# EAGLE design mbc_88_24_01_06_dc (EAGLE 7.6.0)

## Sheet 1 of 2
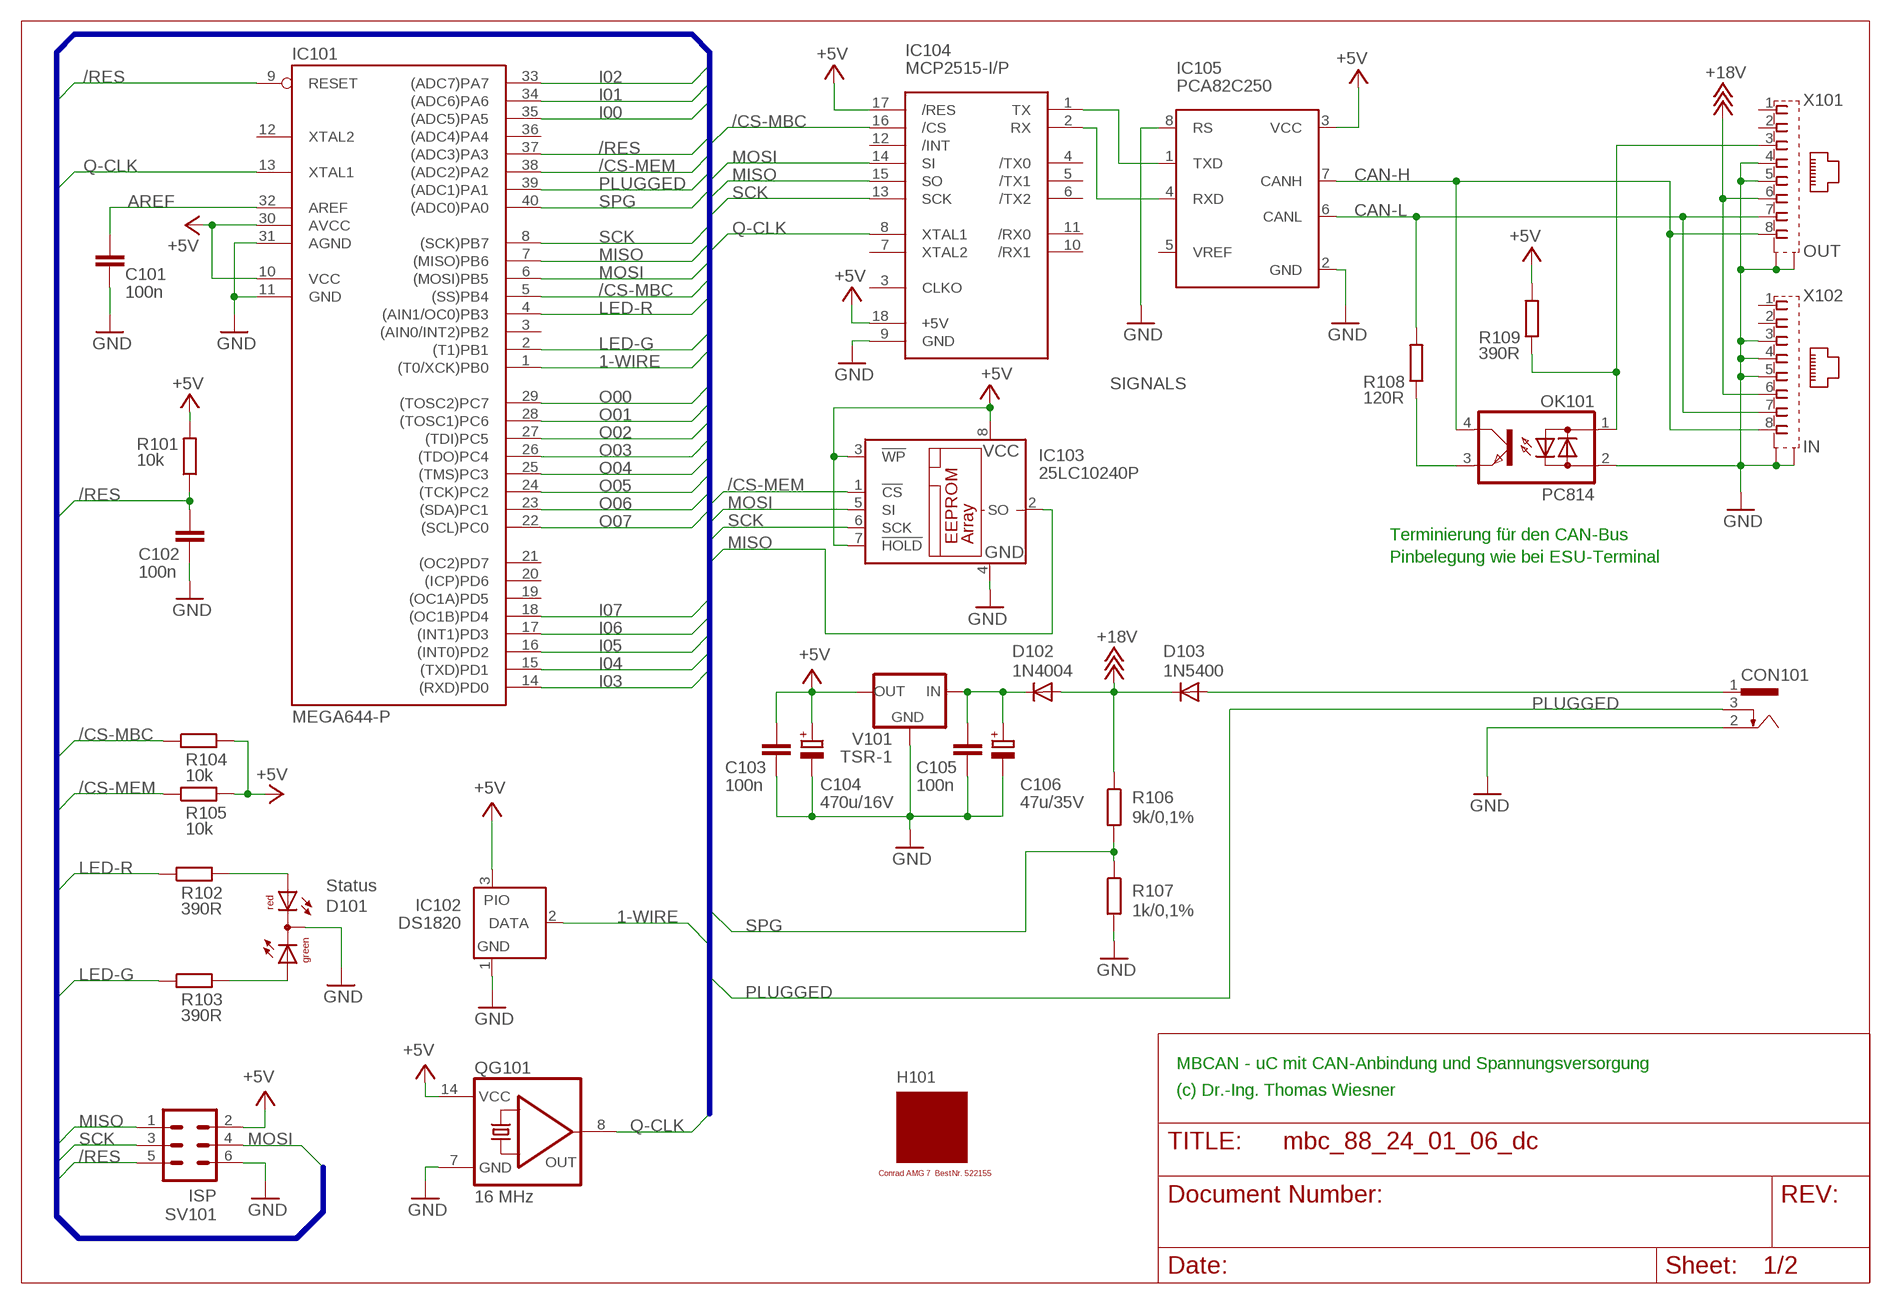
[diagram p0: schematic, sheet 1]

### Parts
C101  100n  C-EU025-025X050  [C025-025X050]
C102  100n  C-EU025-025X050  [C025-025X050]
C103  100n  C-EU025-025X050  [C025-025X050]
C104  470u/16V  CPOL-EUE3.5-8  [E3,5-8]
C105  100n  C-EU025-025X050  [C025-025X050]
C106  47u/35V  CPOL-EUE2.5-7  [E2,5-7]
CON101  POWER-JACK  [POWER-JACK]
D101  Status  DUOLED5MM  [DUOLED5MM]
D102  1N4004  [DO41-10]
D103  1N5400  [DO201-15]
H101  MODULGEHÄUSE-AMG-7  [MODULGEHÄUSE-1]
IC101  MEGA644-P  MEGA323-P  [DIL40]
IC102  DS1820  DS2405  [TO92-]
IC103  25LC10240P  25LC040P  [DIL8]
IC104  MCP2515-I/P  MCP2510-I/P  [DIL18]
IC105  PCA82C250  [DIL08]
OK101  PC814  [DIL04]
QG101  16 MHz  QG5860  [DIL14S]
R101  10k  R-EU_0207/10  [0207/10]
R102  390R  R-EU_0207/10  [0207/10]
R103  390R  R-EU_0207/10  [0207/10]
R104  10k  R-EU_0207/10  [0207/10]
R105  10k  R-EU_0207/10  [0207/10]
R106  9k/0,1%  R-EU_0207/10  [0207/10]
R107  1k/0,1%  R-EU_0207/10  [0207/10]
R108  120R  R-EU_0207/10  [0207/10]
R109  390R  R-EU_0207/10  [0207/10]
SV101  ISP  ML6  [ML6]
V101  TSR-1  [TRACO-TSR-1]
X101  OUT  0446200002  [0446200002]
X102  IN  0446200002  [0446200002]

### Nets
1-WIRE: IC101.1((T0/XCK)PB0) IC102.2(DATA)
+5V: C103.1 C104.+ IC101.10(VCC) IC101.30(AVCC) IC102.3(PIO) IC103.3(!WP) IC103.7(!HOLD) IC103.8(VCC) IC104.17(/RES) IC104.18(+5V) IC105.3(VCC) QG101.14(VCC) R101.2 R104.2 R105.2 R109.2 SV101.2 V101.OUT ; also sheet 2
+18V: D102.A D103.C R106.1 X101.6 X102.6
/CS-MBC: IC101.5((SS)PB4) IC104.16(/CS) R104.1
/CS-MEM: IC101.38((ADC2)PA2) IC103.1(!CS) R105.1
/RES: C102.1 IC101.9(RESET) IC101.37((ADC3)PA3) R101.1 SV101.5
AREF: C101.1 IC101.32(AREF)
CAN-H: IC105.7(CANH) OK101.4(C) X101.8 X102.8
CAN-L: IC105.6(CANL) R108.2 X101.7 X102.7
GND: C101.2 C102.2 C103.2 C104.- C105.2 C106.- CON101.2 D101.K(C) IC101.11(GND) IC101.31(AGND) IC102.1(GND) IC103.4(GND) IC104.9(GND) IC105.2(GND) IC105.8(RS) OK101.2(AC2) QG101.7(GND) R107.2 SV101.6 V101.GND X101.4 X101.5 X101.S@1(S1) X101.S@2(S2) X102.3 X102.4 X102.5 X102.S@1(S1) X102.S@2(S2) ; also sheet 2
I00: IC101.35((ADC5)PA5) ; also sheet 2
I01: IC101.34((ADC6)PA6) ; also sheet 2
I02: IC101.33((ADC7)PA7) ; also sheet 2
I03: IC101.14((RXD)PD0) ; also sheet 2
I04: IC101.15((TXD)PD1) ; also sheet 2
I05: IC101.16((INT0)PD2) ; also sheet 2
I06: IC101.17((INT1)PD3) ; also sheet 2
I07: IC101.18((OC1B)PD4) ; also sheet 2
LED-G: IC101.2((T1)PB1) R103.1
LED-R: IC101.4((AIN1/OC0)PB3) R102.1
MISO: IC101.7((MISO)PB6) IC103.2(SO) IC104.15(SO) SV101.1
MOSI: IC101.6((MOSI)PB5) IC103.5(SI) IC104.14(SI) SV101.4
N$1: IC104.1(TX) IC105.1(TXD)
N$2: IC104.2(RX) IC105.4(RXD)
N$3: OK101.1(AC1) R109.1 X101.3
N$5: OK101.3(E) R108.1
N$6: C105.1 C106.+ D102.C V101.IN
N$9: D101.AR R102.2
N$13: D101.AG R103.2
O00: IC101.29((TOSC2)PC7) ; also sheet 2
O01: IC101.28((TOSC1)PC6) ; also sheet 2
O02: IC101.27((TDI)PC5) ; also sheet 2
O03: IC101.26((TDO)PC4) ; also sheet 2
O04: IC101.25((TMS)PC3) ; also sheet 2
O05: IC101.24((TCK)PC2) ; also sheet 2
O06: IC101.23((SDA)PC1) ; also sheet 2
O07: IC101.22((SCL)PC0) ; also sheet 2
PLUGGED: CON101.3 IC101.39((ADC1)PA1)
Q-CLK: IC101.13(XTAL1) IC104.8(XTAL1) QG101.8(OUT)
SCK: IC101.8((SCK)PB7) IC103.6(SCK) IC104.13(SCK) SV101.3
SPG: IC101.40((ADC0)PA0) R106.2 R107.1
V-NETZTEIL1: CON101.1 D103.A
Unconnected: IC101.3((AIN0/INT2)PB2) IC101.12(XTAL2) IC101.19((OC1A)PD5) IC101.20((ICP)PD6) IC101.21((OC2)PD7) IC101.36((ADC4)PA4) IC104.3(CLKO) IC104.4(/TX0) IC104.5(/TX1) IC104.6(/TX2) IC104.7(XTAL2) IC104.10(/RX1) IC104.11(/RX0) IC104.12(/INT) IC105.5(VREF) X101.1 X101.2 X102.1 X102.2

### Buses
SIGNALS

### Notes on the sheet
- Terminierung für den CAN-Bus
- Pinbelegung wie bei ESU-Terminal
- MBCAN - uC mit CAN-Anbindung und Spannungsversorgung
- (c) Dr.-Ing. Thomas Wiesner

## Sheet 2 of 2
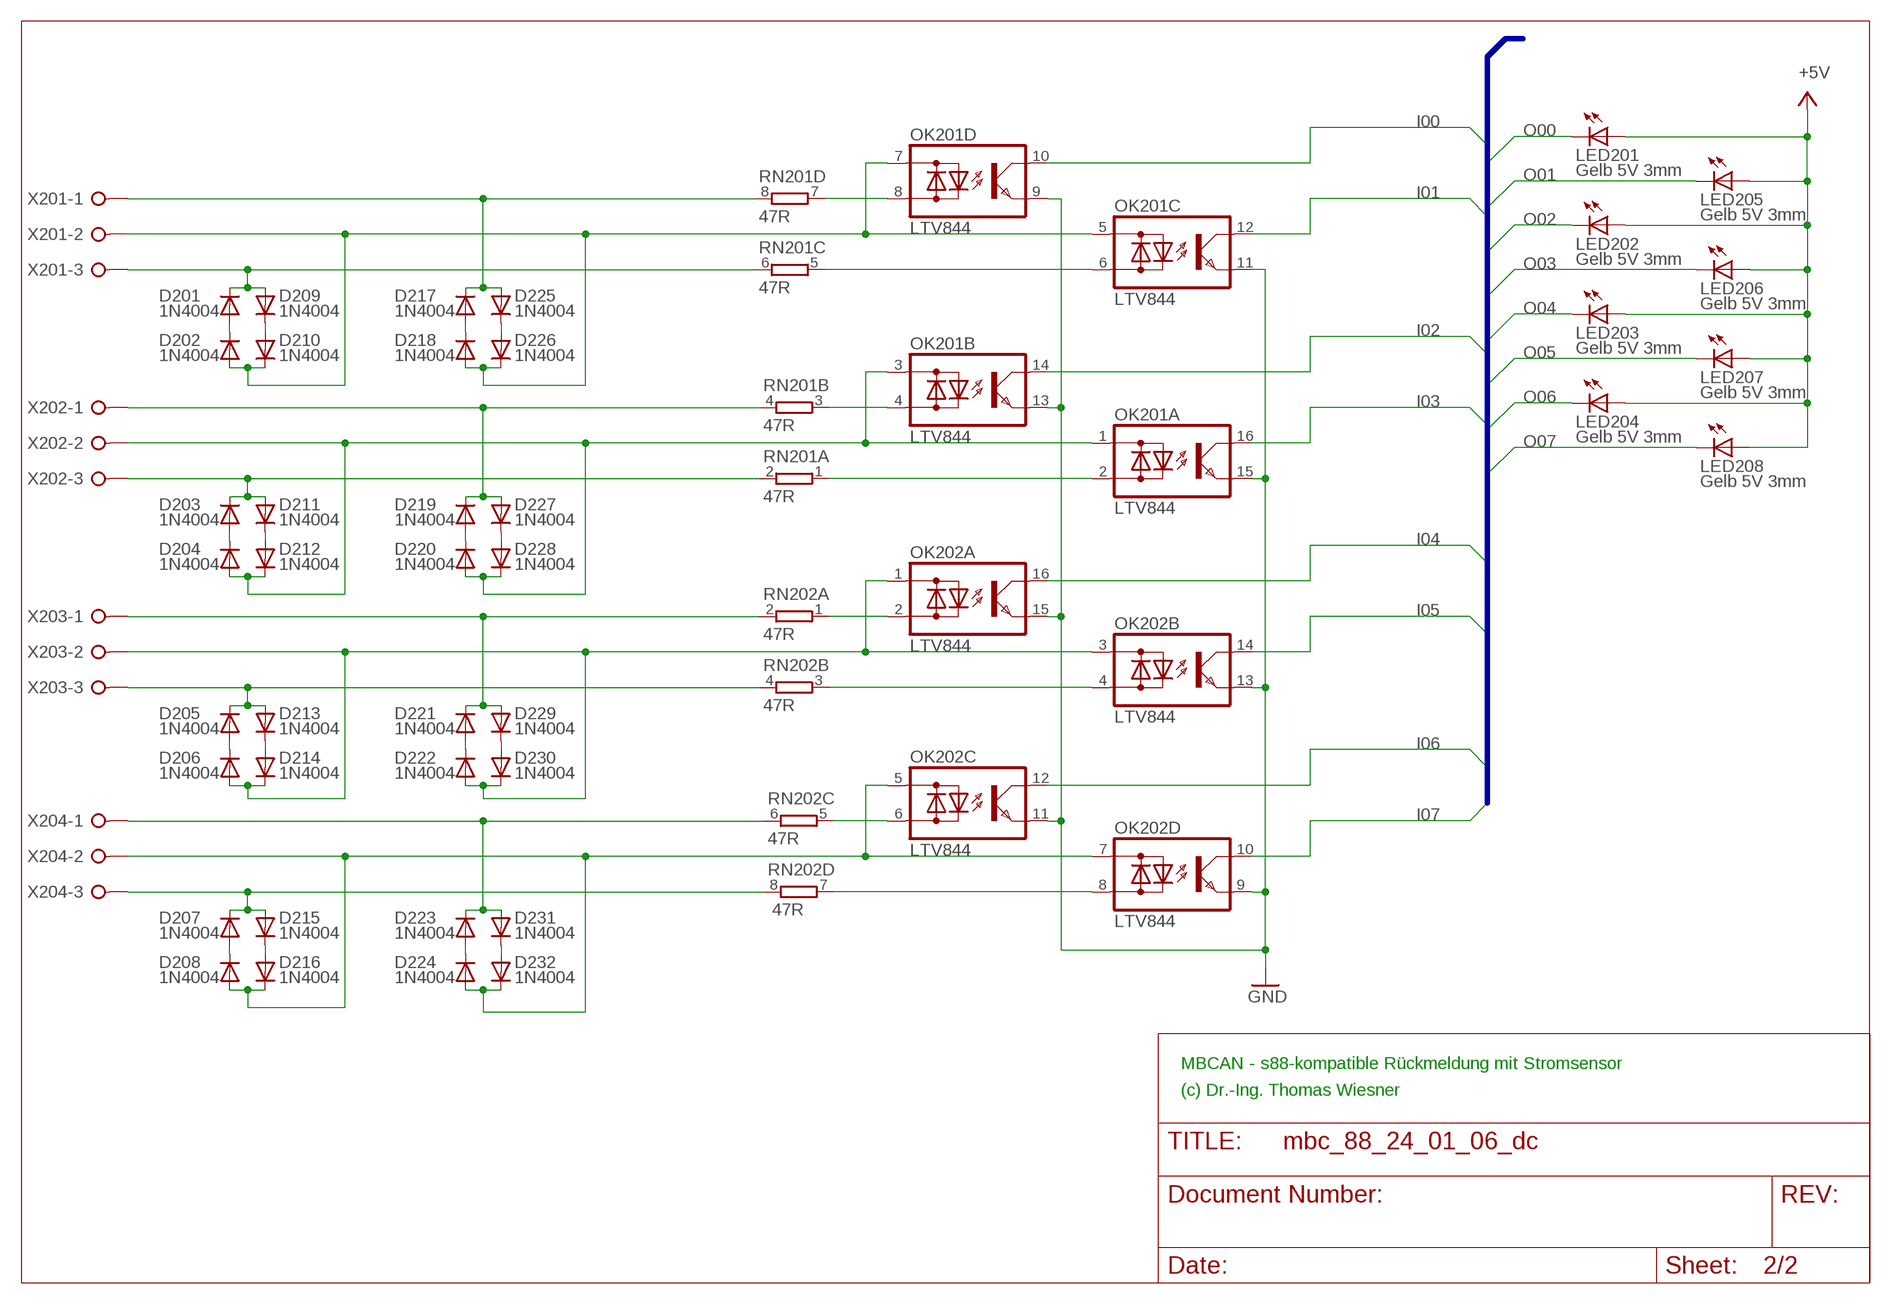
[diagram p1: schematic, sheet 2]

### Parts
D201  1N4004  [DO41-10]
D202  1N4004  [DO41-10]
D203  1N4004  [DO41-10]
D204  1N4004  [DO41-10]
D205  1N4004  [DO41-10]
D206  1N4004  [DO41-10]
D207  1N4004  [DO41-10]
D208  1N4004  [DO41-10]
D209  1N4004  [DO41-10]
D210  1N4004  [DO41-10]
D211  1N4004  [DO41-10]
D212  1N4004  [DO41-10]
D213  1N4004  [DO41-10]
D214  1N4004  [DO41-10]
D215  1N4004  [DO41-10]
D216  1N4004  [DO41-10]
D217  1N4004  [DO41-10]
D218  1N4004  [DO41-10]
D219  1N4004  [DO41-10]
D220  1N4004  [DO41-10]
D221  1N4004  [DO41-10]
D222  1N4004  [DO41-10]
D223  1N4004  [DO41-10]
D224  1N4004  [DO41-10]
D225  1N4004  [DO41-10]
D226  1N4004  [DO41-10]
D227  1N4004  [DO41-10]
D228  1N4004  [DO41-10]
D229  1N4004  [DO41-10]
D230  1N4004  [DO41-10]
D231  1N4004  [DO41-10]
D232  1N4004  [DO41-10]
LED201  Gelb 5V 3mm  LED3MM  [LED3MM]
LED202  Gelb 5V 3mm  LED3MM  [LED3MM]
LED203  Gelb 5V 3mm  LED3MM  [LED3MM]
LED204  Gelb 5V 3mm  LED3MM  [LED3MM]
LED205  Gelb 5V 3mm  LED3MM  [LED3MM]
LED206  Gelb 5V 3mm  LED3MM  [LED3MM]
LED207  Gelb 5V 3mm  LED3MM  [LED3MM]
LED208  Gelb 5V 3mm  LED3MM  [LED3MM]
OK201  LTV844  TIL196  [DIL16]
OK202  LTV844  TIL196  [DIL16]
RN201  47R  E4R  [SIL8]
RN202  47R  E4R  [SIL8]
X201  W237-03P  [W237-133]
X202  W237-03P  [W237-133]
X203  W237-03P  [W237-133]
X204  W237-03P  [W237-133]

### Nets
+5V: LED201.A LED202.A LED203.A LED204.A LED205.A LED206.A LED207.A LED208.A ; also sheet 1
GND: OK201.9(D:E) OK201.11(C:E) OK201.13(B:E) OK201.15(A:E) OK202.9(D:E) OK202.11(C:E) OK202.13(B:E) OK202.15(A:E) ; also sheet 1
I00: OK201.10(D:C) ; also sheet 1
I01: OK201.12(C:C) ; also sheet 1
I02: OK201.14(B:C) ; also sheet 1
I03: OK201.16(A:C) ; also sheet 1
I04: OK202.16(A:C) ; also sheet 1
I05: OK202.14(B:C) ; also sheet 1
I06: OK202.12(C:C) ; also sheet 1
I07: OK202.10(D:C) ; also sheet 1
N$11: D201.A D202.C
N$12: D201.C D209.A RN201.6 X201.3
N$15: D217.A D218.C
N$16: D225.C D226.A
N$17: D217.C D225.A RN201.8 X201.1
N$18: D202.A D210.C D218.A D226.C OK201.5(C:AC1) OK201.7(D:AC1) X201.2
N$19: D203.A D204.C
N$20: D209.C D210.A
N$21: D211.C D212.A
N$22: D203.C D211.A RN201.2 X202.3
N$31: D219.A D220.C
N$32: D227.C D228.A
N$33: D219.C D227.A RN201.4 X202.1
N$34: D204.A D212.C D220.A D228.C OK201.1(A:AC1) OK201.3(B:AC1) X202.2
N$35: D205.A D206.C
N$36: D213.C D214.A
N$37: D205.C D213.A RN202.4 X203.3
N$39: D221.A D222.C
N$40: D229.C D230.A
N$41: D221.C D229.A RN202.2 X203.1
N$42: OK202.8(D:AC2) RN202.7
N$43: OK202.6(C:AC2) RN202.5
N$44: OK202.4(B:AC2) RN202.3
N$45: OK202.2(A:AC2) RN202.1
N$46: OK201.2(A:AC2) RN201.1
N$48: OK201.4(B:AC2) RN201.3
N$49: D206.A D214.C D222.A D230.C OK202.1(A:AC1) OK202.3(B:AC1) X203.2
N$50: D207.A D208.C
N$51: D215.C D216.A
N$52: D207.C D215.A RN202.8 X204.3
N$54: D223.A D224.C
N$55: D231.C D232.A
N$56: D223.C D231.A RN202.6 X204.1
N$57: D208.A D216.C D224.A D232.C OK202.5(C:AC1) OK202.7(D:AC1) X204.2
N$64: OK201.6(C:AC2) RN201.5
N$65: OK201.8(D:AC2) RN201.7
O00: LED201.K(C) ; also sheet 1
O01: LED205.K(C) ; also sheet 1
O02: LED202.K(C) ; also sheet 1
O03: LED206.K(C) ; also sheet 1
O04: LED203.K(C) ; also sheet 1
O05: LED207.K(C) ; also sheet 1
O06: LED204.K(C) ; also sheet 1
O07: LED208.K(C) ; also sheet 1

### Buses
B$1

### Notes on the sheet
- MBCAN - s88-kompatible Rückmeldung mit Stromsensor
- (c) Dr.-Ing. Thomas Wiesner

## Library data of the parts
C101-C103 C105 = rcl:C-EU: CAPACITOR, European symbol
C104 C106 = rcl:CPOL-EU: POLARIZED CAPACITOR, European symbol
CON101 = mbc:POWER-JACK: Power-Stecker für 2,5 mm Hohlbuchse
D101 = led:DUOLED5MM: DUO LED 2 colors, 5 mm, round
D102 D201-D232 = diode:1N4004: DIODE
D103 = diode:1N5400: DIODE
H101 = mbc:MODULGEHÄUSE-AMG-7: Gehäuse
IC101 = atmel:MEGA323-P: MICROCONTROLLER 32 Kbytes FLASH 2 Kbytes SRAM 1 Kbytes EEPROM USART 8-channel 10 bit ADC Source: avr.lbr; OC_FARNELL: unknown; OC_NEWARK: unknown
IC102 = maxim:DS2405: Addressable Switch DALLAS Semiconductor; MF: DALLAS SEMICONDUCTOR; MPN: DS2405; OC_FARNELL: 1188025; OC_NEWARK: 06F4645
IC103 = microchip:25*: Serial EEPROM 4K/ 8K , SPI bus; MF: MICROCHIP; MPN: 25LC040/P; OC_FARNELL: 9758100; OC_NEWARK: 96K4091
IC104 = mbc:MCP2510: BASIC-CAN 2.0a Controller Stand-alone CAN controller von Microchip
IC105 = micro-philips:PCA82C250: CAN CONTROLLER INTERFACE; OC_FARNELL: 3692358; OC_NEWARK: unknown
LED201-LED208 = led:LED: LED
OK101 = optocoupler:PC814: SHARP OPTO COUPLER; OC_FARNELL: 9707662; OC_NEWARK: unknown
OK201 OK202 = optocoupler:TIL196: TEXAS INSTRUMENTS OPTO COUPLER; MPN: TIL 196; OC_FARNELL: 1683367; OC_NEWARK: 05R6476
QG101 = crystal:QG5860: CRYSTAL RESONATOR; OC_FARNELL: unknown; OC_NEWARK: unknown
R101-R109 = resistor:R-EU_: RESISTOR, European symbol
RN201 RN202 = resistor-sil:E4R: SIL RESISTOR; OC_FARNELL: unknown; OC_NEWARK: unknown
SV101 = con-ml:ML6: HARTING; OC_FARNELL: unknown; OC_NEWARK: unknown
V101 = mbc:TSR-1: Spannungsregler Hersteller: TRACO Typ: TSR-1 5V: TSR 1-2450 Spg: 5V Strom: 1A Reichelt TSR 1-2450
X101 X102 = mbc:0446200002: RJ-45 INVERTED MODULAR JACK ASSEMBLY WITH RJ-11 KEEPOUT FEATURE Source: Data sheet MOLEX 0446200002 BUCHSE, RJ45, GESCHIRMT Source: Farnell; MF: MOLEX; MPN: 0446200002; OC_FARNELL: 9251910
X201-X204 = con-wago-508:W237-03P: WAGO SREW CLAMP; OC_FARNELL: unknown; OC_NEWARK: unknown

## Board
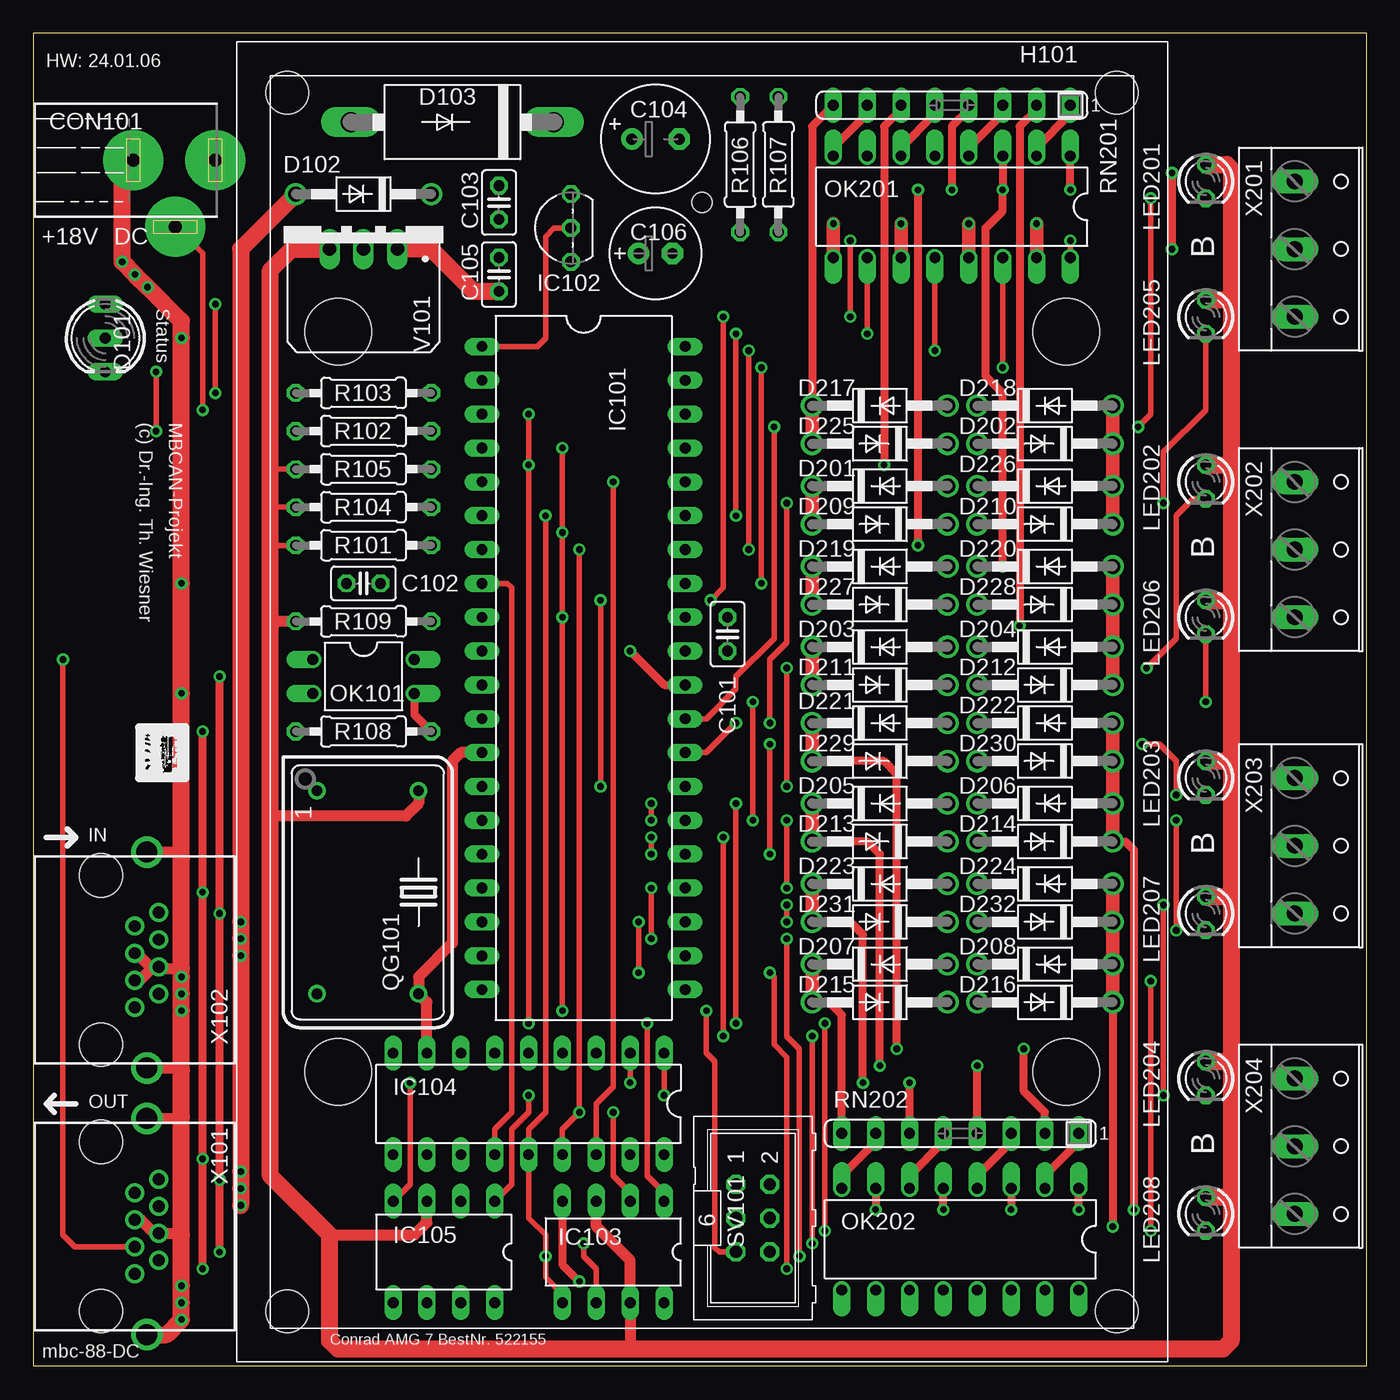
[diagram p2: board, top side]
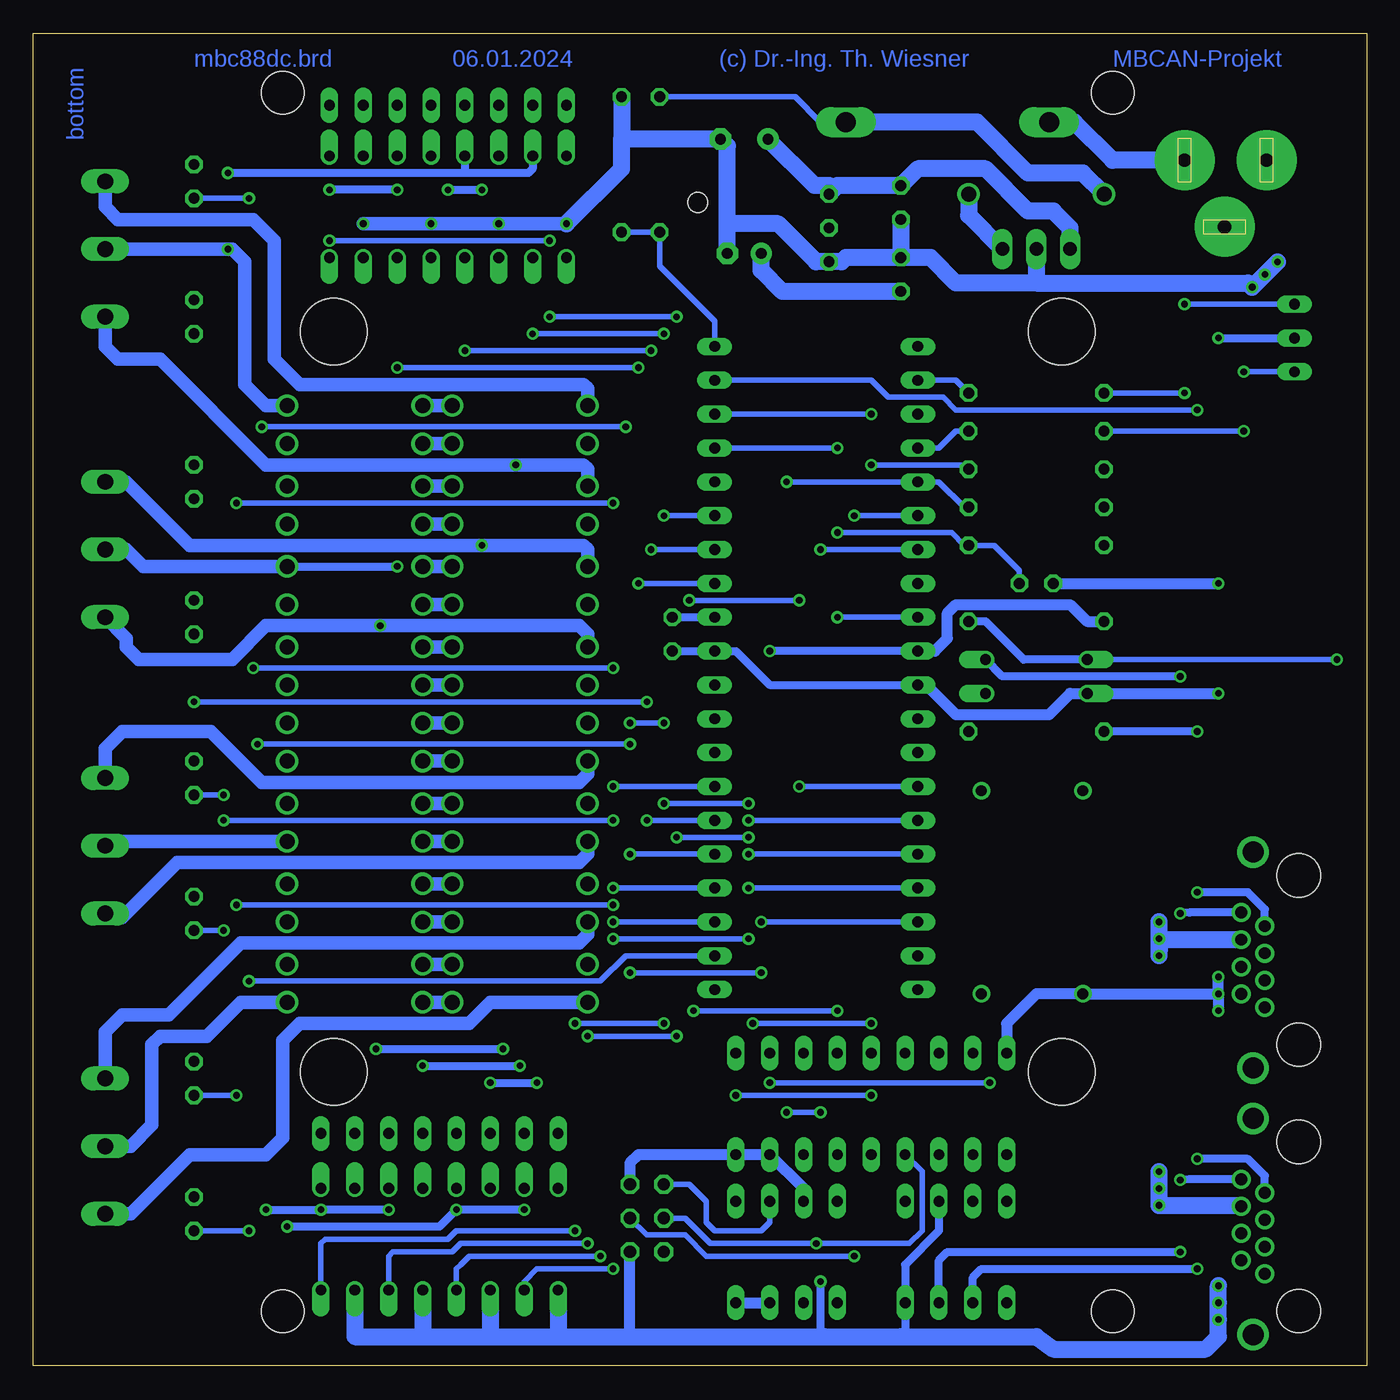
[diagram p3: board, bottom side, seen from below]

Size 100 x 99.99 mm. Coordinates in mm from the lower left corner, seen from the top.
Outline: 0,99.99 0,0 100,0 100,99.99 0,99.99
Copper layers (1*16): Top 0.035mm / dielectric 1.5mm / Bottom 0.035mm
Design rules "default *": minimum track width 10mil, minimum drill 0.5mm, track to track 8mil, track to pad 8mil, pad to pad 8mil, via to via 8mil, smd to smd 8mil, copper to edge 40mil, drill to drill 8mil, minimum pad ring 10mil, minimum via ring 8mil, stop-mask expansion 4mil, vias tented up to drill 0mil, thermal gap 10mil

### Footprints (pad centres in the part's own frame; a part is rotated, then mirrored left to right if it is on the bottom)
C025-025X050 = drill 0.813 octagon: 1 -1.27,0; 2 1.27,0
E3,5-8 = drill 0.813 pad 1.6: + -1.778,0 | drill 0.813 pad 1.6 octagon: - 1.778,0
E2,5-7 = drill 0.813 pad 1.6: + -1.27,0 | drill 0.813 pad 1.6 octagon: - 1.27,0
POWER-JACK = drill 1 pad 4.5: 1 0,6.03; 2 0,-0.12; 3 5,3.03
DUOLED5MM = drill 0.813 long: AG -2.54,0; AR 2.54,0; K 0,0
DO41-10 = drill 1.118: A 5.08,0; C -5.08,0
DO201-15 = drill 1.499 long: A 7.62,0; C -7.62,0
MODULGEHÄUSE-1 = hole 3.2: -45.72,-31.115; -45.72,31.115; 45.72,31.115; 45.72,-31.115 | hole 5: -27.781,-27.305; 27.781,-27.305; -27.781,27.305; 27.781,27.305 | hole 1.5: -37.465,0
DIL40 = drill 0.813 long: 1 -24.13,-7.62; 2 -21.59,-7.62; 3 -19.05,-7.62; 4 -16.51,-7.62; 5 -13.97,-7.62; 6 -11.43,-7.62; 7 -8.89,-7.62; 8 -6.35,-7.62; 9 -3.81,-7.62; 10 -1.27,-7.62; 11 1.27,-7.62; 12 3.81,-7.62; 13 6.35,-7.62; 14 8.89,-7.62; 15 11.43,-7.62; 16 13.97,-7.62; 17 16.51,-7.62; 18 19.05,-7.62; 19 21.59,-7.62; 20 24.13,-7.62; 21 24.13,7.62; 22 21.59,7.62; 23 19.05,7.62; 24 16.51,7.62; 25 13.97,7.62; 26 11.43,7.62; 27 8.89,7.62; 28 6.35,7.62; 29 3.81,7.62; 30 1.27,7.62; 31 -1.27,7.62; 32 -3.81,7.62; 33 -6.35,7.62; 34 -8.89,7.62; 35 -11.43,7.62; 36 -13.97,7.62; 37 -16.51,7.62; 38 -19.05,7.62; 39 -21.59,7.62; 40 -24.13,7.62
TO92- = drill 0.813 octagon: 1 -2.54,0; 2 0,0; 3 2.54,0
DIL8 = drill 0.813 long: 1 -3.81,-3.81; 2 -1.27,-3.81; 3 1.27,-3.81; 4 3.81,-3.81; 5 3.81,3.81; 6 1.27,3.81; 7 -1.27,3.81; 8 -3.81,3.81
DIL18 = drill 0.813 long: 1 -10.16,-3.81; 2 -7.62,-3.81; 3 -5.08,-3.81; 4 -2.54,-3.81 | drill 0.8 long: 5 0,-3.81; 6 2.54,-3.81; 7 5.08,-3.81; 8 7.62,-3.81; 9 10.16,-3.81; 10 10.16,3.81; 11 7.62,3.81; 12 5.08,3.81; 13 2.54,3.81; 14 0,3.81; 15 -2.54,3.81; 16 -5.08,3.81; 17 -7.62,3.81; 18 -10.16,3.81
DIL08 = drill 0.813 long: 1 -3.81,-3.81; 2 -1.27,-3.81; 3 1.27,-3.81; 4 3.81,-3.81; 5 3.81,3.81; 6 1.27,3.81; 7 -1.27,3.81; 8 -3.81,3.81
LED3MM = drill 0.813 octagon: A -1.27,0; K 1.27,0
DIL04 = drill 0.813 offset: 1 -1.27,-3.81; 2 1.27,-3.81; 3 1.27,3.81; 4 -1.27,3.81
DIL16 = drill 0.813 offset: 1 -8.89,-3.81; 2 -6.35,-3.81; 3 -3.81,-3.81; 4 -1.27,-3.81; 5 1.27,-3.81; 6 3.81,-3.81; 7 6.35,-3.81; 8 8.89,-3.81; 9 8.89,3.81; 10 6.35,3.81; 11 3.81,3.81; 12 1.27,3.81; 13 -1.27,3.81; 14 -3.81,3.81; 15 -6.35,3.81; 16 -8.89,3.81
DIL14S = drill 0.813: 1 -7.62,-3.81; 7 7.62,-3.81; 8 7.62,3.81; 14 -7.62,3.81
0207/10 = drill 0.813 octagon: 1 -5.08,0; 2 5.08,0
SIL8 = drill 0.813 long: 1 -8.89,0; 2 -6.35,0; 3 -3.81,0; 4 -1.27,0; 5 1.27,0; 6 3.81,0; 7 6.35,0; 8 8.89,0
ML6 = drill 0.914 octagon: 1 -2.54,-1.27; 2 -2.54,1.27; 3 0,-1.27; 4 0,1.27; 5 2.54,-1.27; 6 2.54,1.27
TRACO-TSR-1 = drill 1.016 long: GND 0,2.54; IN -2.54,2.54; OUT 2.54,2.54
0446200002 = drill 0.889 pad 1.422: 1 3.556,2.54; 2 2.54,4.318; 3 1.524,2.54; 4 0.508,4.318; 5 -0.508,2.54; 6 -1.524,4.318; 7 -2.54,2.54; 8 -3.556,4.318 | drill 1.575 pad 2.286: S@1 -8.103,3.429; S@2 8.103,3.429 | hole 3.251: 6.35,0; -6.35,0
W237-133 = drill 1.194 long: 1 -5.08,-0.635; 2 0,-0.635; 3 5.08,-0.635

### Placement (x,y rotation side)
C101  52.07,54.91 270 top
C102  24.77,58.72 180 top
C103  34.92,87.29 270 top
C104  46.67,92.06 0 top
C105  34.92,81.9 90 top
C106  46.67,83.48 0 top
CON101  7.62,90.47 270 top
D101  5.4,77.13 270 top
D102  24.77,87.93 180 top
D103  31.43,93.33 180 top
D201  63.5,66.02 0 top
D202  75.88,66.02 0 top
D203  63.5,53.95 0 top
D204  75.88,53.95 0 top
D205  63.5,42.21 0 top
D206  75.88,42.21 0 top
D207  63.5,30.14 0 top
D208  75.88,30.14 0 top
D209  63.5,63.16 180 top
D210  75.88,63.16 180 top
D211  63.5,51.1 180 top
D212  75.88,51.1 180 top
D213  63.5,39.35 180 top
D214  75.88,39.35 180 top
D215  63.5,27.29 180 top
D216  75.88,27.29 180 top
D217  63.5,72.05 0 top
D218  75.88,72.05 0 top
D219  63.5,59.99 0 top
D220  75.88,59.99 0 top
D221  63.5,48.24 0 top
D222  75.88,48.24 0 top
D223  63.5,36.17 0 top
D224  75.88,36.17 0 top
D225  63.5,69.2 180 top
D226  75.88,69.2 180 top
D227  63.5,57.13 180 top
D228  75.88,57.13 180 top
D229  63.5,45.38 180 top
D230  75.88,45.38 180 top
D231  63.5,33.32 180 top
D232  75.88,33.32 180 top
H101  50.16,49.83 270 top
IC101  41.27,52.37 270 top
IC102  40.32,85.39 90 top
IC103  43.5,8.55 180 top
IC104  37.15,19.66 180 top
IC105  30.8,8.55 180 top
LED201  87.95,88.88 270 top
LED202  87.95,66.34 270 top
LED203  87.95,44.11 270 top
LED204  87.95,21.57 270 top
LED205  87.95,78.72 270 top
LED206  87.95,56.18 270 top
LED207  87.95,33.95 270 top
LED208  87.95,11.41 270 top
OK101  24.77,51.73 270 top
OK201  68.9,86.98 180 top
OK202  69.53,9.51 180 top
QG101  25.08,35.54 270 top
R101  24.77,61.57 180 top
R102  24.77,70.15 180 top
R103  24.77,73.01 180 top
R104  24.77,64.43 180 top
R105  24.77,67.29 180 top
R106  53.02,90.15 270 top
R107  55.88,90.15 90 top
R108  24.77,47.6 180 top
R109  24.77,55.86 180 top
RN201  68.9,94.59 180 top
RN202  69.53,17.44 180 top
SV101  53.98,11.09 270 top
V101  24.77,86.34 180 top
X101  5.08,10.46 270 top
X102  5.08,30.46 270 top
X201  95.25,83.8 270 top
X202  95.25,61.26 270 top
X203  95.25,39.03 270 top
X204  95.25,16.49 270 top

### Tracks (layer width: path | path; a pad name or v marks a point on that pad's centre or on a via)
1-WIRE
  Top 0.406: IC102.2 39.05,85.39 38.42,84.75 38.42,77.13 37.78,76.5 IC101.1
+5V  (via drill 0.5)
  Top 0.406: R105.2 17.78,67.29 | R104.2 17.78,64.43 | R101.2 17.78,61.57 | 18.1,55.86 17.78,55.54
  Top 0.61: v44.77,53.64 47.31,51.1 IC101.30
  Top 0.813: R109.2 18.1,55.86 | QG101.14 28.89,42.21 27.94,41.25 17.78,41.25 | IC103.3 42.23,10.46 44.77,7.92 IC103.7 44.77,1.25 | 22.23,9.82 28.57,9.82 29.53,10.78 IC105.3
  Top 1.016: 89.53,22.84 89.85,22.52 | 89.53,45.38 89.85,45.06 | 89.85,13 89.85,12.36 89.53,12.68 89.85,13
  Top 1.27: LED201.A 89.53,90.15 89.85,89.83 89.85,79.99 | 89.85,79.99 89.85,67.61 | 89.85,67.61 89.85,57.45 | 89.85,57.45 89.85,45.06 89.85,35.22 | 89.85,35.22 89.85,22.52 89.85,13 | LED204.A 89.53,22.84 | LED207.A 89.85,35.22 | LED203.A 89.53,45.38 | LED206.A 89.85,57.45 | LED202.A 89.85,67.61 | LED205.A 89.85,79.99 | LED208.A 89.53,12.68 | 89.85,12.36 89.85,1.89 89.22,1.25 44.77,1.25 22.86,1.25 22.23,1.89 22.23,9.82 17.78,14.27 17.78,41.25 17.78,55.54 17.78,61.57 17.78,64.43 17.78,67.29 17.78,82.21 19.37,83.8 V101.OUT
  Bottom 0.61: IC101.10 v44.77,53.64
  Bottom 0.813: IC101.10 32.38,53.64 31.43,54.59 31.43,56.49 30.8,57.13 22.23,57.13 20.95,55.86 R109.2 | SV101.2 55.24,15.22 54.61,15.86 IC104.18 IC104.17 42.23,13.32 IC103.3 | IC103.8 IC103.7
  Bottom 1.27: C104.+ 41.4,88.56 40.32,88.56 IC102.3 39.69,88.56 C103.1 33.66,89.83 28.57,89.83 25.4,86.66 23.5,86.66 22.23,85.39 V101.OUT
+18V  (via drill 0.5)
  Top 1.27: D102.A 15.56,83.8 v15.56,33.32 v15.56,32.05 v15.56,30.78 v15.56,14.59 v15.56,13.32 v15.56,12.04
  Bottom 0.406: D103.C 40.96,93.33 42.86,95.23 R106.1
  Bottom 1.27: D102.A 21.27,89.52 25.4,89.52 29.21,93.33 D103.C | X101.6 9.46,12.04 v15.56,12.04 v15.56,14.59 | X102.6 15.49,31.98 v15.56,32.05 | v15.56,32.05 15.56,32.68 | v15.56,32.05 15.56,31.09 | v15.56,30.78 v15.56,33.32
/CS-MBC  (via drill 0.5)
  Top 0.406: IC104.16 42.23,19.66 43.5,20.93 v43.5,66.34
  Bottom 0.406: v43.5,66.34 IC101.5 32.07,66.34 30.16,64.43 R104.1
/CS-MEM  (via drill 0.5)
  Top 0.406: IC103.1 47.31,13 46.04,14.27 v46.04,25.7 | v37.15,25.7 v37.15,67.61 v37.15,71.42
  Bottom 0.406: v46.04,25.7 v37.15,25.7 | v37.15,67.61 30.16,67.61 R105.1 | IC101.38 v37.15,71.42
/RES  (via drill 0.5)
  Top 0.406: SV101.5 51.44,8.55 51.12,8.87 51.12,22.84 50.48,23.48 v50.48,26.65 | v39.69,26.65 v39.69,56.18 v39.69,62.53 v39.69,68.88
  Bottom 0.406: v50.48,26.65 v39.69,26.65 | v39.69,56.18 IC101.9 | v39.69,62.53 31.11,62.53 30.16,61.57 R101.1 27.94,61.57 26.04,59.67 C102.1 | IC101.37 v39.69,68.88
AREF
  Bottom 0.61: C101.1 IC101.32
CAN-H  (via drill 0.5)
  Top 0.61: v13.97,8.55 v13.97,13.95 v13.97,33.95 v13.97,51.73
  Bottom 0.61: IC105.7 32.07,7.92 31.43,8.55 v13.97,8.55 | v13.97,51.73 27.3,51.73 OK101.4 | X102.8 13.27,34.02 v13.97,33.95 | X101.8 13.27,14.01 v13.97,13.95
CAN-L  (via drill 0.5)
  Top 0.61: v12.7,7.28 v12.7,15.54 v12.7,35.54 v12.7,47.6
  Bottom 0.61: IC105.6 29.53,6.65 28.89,7.28 v12.7,7.28 | v12.7,47.6 R108.2 | X102.7 7.62,34.27 8.89,35.54 v12.7,35.54 | X101.7 7.62,14.27 8.89,15.54 v12.7,15.54
GND  (via drill 0.5)
  Top 0.61: IC103.4 39.69,7.6 v40.96,6.33
  Top 0.813: X102.S@1 10.63,38.56 11.11,38.08 | X102.S@2 10.96,22.36 11.11,22.21 | X101.S@1 10.96,18.56 11.11,18.71 | X101.5 8.06,10.97 8.89,10.14 9.21,10.14 X101.4 10.99,9.95 11.11,9.82 | X102.5 7.75,30.97 8.89,29.82 | 8.89,29.82 9.27,29.82 | 9.27,29.82 X102.4 | X102.3 8,28.94 8.89,29.82 | 9.27,29.82 11.11,29.82
  Top 1.016: OK201.15 v75.25,85.7 | OK201.13 v70.17,85.7 | OK201.11 v65.09,85.7 | OK201.9 v60.01,85.7
  Top 1.27: X101.S@2 9.99,2.35 v11.11,3.47 v11.11,4.74 v11.11,6.01 11.11,9.82 11.11,18.71 11.11,22.21 v11.11,26.65 v11.11,27.92 v11.11,29.19 11.11,29.82 11.11,38.08 v11.11,50.46 v11.11,58.72 v11.11,77.13 11.11,78.4 v8.57,80.94 v7.62,81.9 v6.67,82.85 6.67,89.64 CON101.2
  Bottom 0.61: v11.11,77.13 D101.K | C101.2 IC101.31 47.31,53.64 44.77,51.1 IC101.11 | 34.92,2.2 34.61,2.52 IC105.8 34.61,7.6 32.07,10.14 IC105.2 | v40.96,6.33 40.96,2.52 40.64,2.2
  Bottom 0.813: 55.24,2.2 SV101.6 | C102.2 v11.11,58.72 | v11.11,27.92 QG101.7 24.77,27.92 26.99,25.7 IC104.9 | v11.11,27.92 v11.11,29.19 | v11.11,27.92 v11.11,26.65 | v11.11,50.46 OK101.2 22.23,50.46 23.81,48.88 30.8,48.88 33.02,51.1 IC101.11
  Bottom 1.016: v75.25,85.7 v70.17,85.7 v65.09,85.7 v60.01,85.7
  Bottom 1.27: C106.- 47.94,85.7 | 47.94,85.7 47.94,91.55 C104.- 55.88,92.06 | R107.2 55.88,92.06 | v60.01,85.7 55.88,89.83 55.88,92.06 | C103.2 C105.2 | C105.2 39.05,83.17 39.37,82.85 IC102.1 41.27,82.85 44.13,85.7 47.94,85.7 | V101.GND 24.77,81.26 | 24.77,81.26 30.8,81.26 32.7,83.17 C105.2 | OK202.15 75.88,2.2 70.8,2.2 | 70.8,2.2 65.72,2.2 | 65.72,2.2 60.64,2.2 | 60.64,2.2 55.24,2.2 40.64,2.2 34.92,2.2 24.77,2.2 23.5,1.25 12.06,1.25 11.11,2.2 v11.11,3.47 v11.11,4.74 v11.11,6.01 | OK202.9 60.64,2.2 | OK202.11 65.72,2.2 | OK202.13 70.8,2.2 | 24.77,81.26 8.89,81.26 v8.57,80.94 v7.62,81.9 v6.67,82.85
I00  (via drill 0.5)
  Top 0.406: v52.7,63.8 v52.7,77.45 | v62.55,77.45 OK201.10
  Bottom 0.406: IC101.35 v52.7,63.8 | v52.7,77.45 v62.55,77.45
I01  (via drill 0.5)
  Top 0.406: v53.66,61.26 v53.66,76.18 | v67.63,76.18 OK201.12
  Bottom 0.406: IC101.34 v53.66,61.26 | v53.66,76.18 v67.63,76.18
I02  (via drill 0.5)
  Top 0.406: v54.61,58.72 v54.61,74.91 | v72.71,74.91 OK201.14
  Bottom 0.406: IC101.33 v54.61,58.72 | v54.61,74.91 v72.71,74.91
I03  (via drill 0.5)
  Top 0.406: OK201.16 v77.79,84.44 | v61.28,84.44 v61.28,78.72 | v51.75,78.72 51.75,58.4 v50.8,57.45 | v42.55,57.45 v42.55,43.48
  Bottom 0.406: v77.79,84.44 v61.28,84.44 | v61.28,78.72 v51.75,78.72 | v50.8,57.45 v42.55,57.45 | v42.55,43.48 IC101.14
I04  (via drill 0.5)
  Top 0.406: v59.37,10.14 v59.37,25.7 | v52.7,25.7 v52.7,42.21 | v46.35,42.21 v46.35,40.94
  Bottom 0.406: OK202.16 78.42,9.19 78.11,9.51 68.9,9.51 68.26,10.14 v59.37,10.14 | v59.37,25.7 v52.7,25.7 | v52.7,42.21 v46.35,42.21 | v46.35,40.94 IC101.15
I05  (via drill 0.5)
  Top 0.406: v58.42,9.19 v58.42,24.75 | v51.75,24.75 v51.75,39.67 | v46.35,39.67 v46.35,38.4
  Bottom 0.406: OK202.14 73.34,8.24 73.03,8.55 68.58,8.55 67.94,9.19 v58.42,9.19 | v58.42,24.75 v51.75,24.75 | v51.75,39.67 v46.35,39.67 | v46.35,38.4 IC101.16
I06  (via drill 0.5)
  Top 0.406: v57.47,8.24 57.47,23.79 56.52,24.75 v56.52,32.05 | v46.35,32.05 v46.35,35.86
  Bottom 0.406: OK202.12 68.26,7.28 67.94,7.6 67.31,8.24 v57.47,8.24 | v56.52,32.05 v46.35,32.05 | v46.35,35.86 IC101.17
I07  (via drill 0.5)
  Top 0.406: v56.52,7.28 56.52,23.16 55.56,24.11 55.56,29.19 v55.24,29.51 | v45.4,29.51 v45.4,33.32
  Bottom 0.406: OK202.10 63.18,6.33 62.23,7.28 v56.52,7.28 | v55.24,29.51 v45.4,29.51 | v45.4,33.32 IC101.18
LED-G
  Bottom 0.406: IC101.2 30.8,73.96 R103.1
LED-R
  Bottom 0.406: R102.1 30.8,70.15 32.07,68.88 IC101.4
MISO  (via drill 0.5)
  Top 0.406: IC104.15 39.69,17.76 v40.96,19.03 v40.96,61.26 | IC103.2 44.77,13 43.5,14.27 v43.5,19.03
  Bottom 0.406: v40.96,61.26 IC101.7 | v43.5,19.03 v40.96,19.03 | SV101.1 50.8,13.63 49.53,12.36 49.53,10.78 48.9,10.14 45.4,10.14 44.77,10.78 IC103.2
MOSI  (via drill 0.5)
  Top 0.406: v38.42,63.8 38.42,19.03 37.15,17.76 IC104.14 37.15,11.09 38.42,9.82 v38.42,8.24 38.42,6.65 39.69,5.38 IC103.5
  Bottom 0.406: v38.42,63.8 IC101.6 | SV101.4 53.98,9.82 51.12,9.82 49.53,8.24 v38.42,8.24
N$1  (via drill 0.5)
  Top 0.406: IC104.1 v47.31,20.3 | v37.15,20.3 37.15,19.03 35.88,17.76 35.88,13.63 IC105.1
  Bottom 0.406: v47.31,20.3 v37.15,20.3
N$2  (via drill 0.5)
  Top 0.406: IC104.2 v44.77,21.25 | v28.26,21.25 28.26,13.63 IC105.4
  Bottom 0.406: v44.77,21.25 v28.26,21.25
N$3  (via drill 0.5)
  Top 0.406: X101.3 3.11,8.93 2.22,9.82 v2.22,53
  Bottom 0.406: v2.22,53 OK101.1
  Bottom 0.61: OK101.1 25.72,53 28.57,55.86 R109.1
N$5
  Top 0.61: OK101.3 28.57,48.88 R108.1
N$6
  Top 1.27: C105.1 33.02,80.62 29.84,83.8 V101.IN
  Bottom 1.27: D102.C 29.84,86.34 V101.IN | C105.1 43.81,80.62 45.4,82.21 C106.+
N$9  (via drill 0.5)
  Top 0.406: v9.21,74.59 v9.21,70.15
  Bottom 0.406: D101.AR v9.21,74.59 | v9.21,70.15 R102.2
N$11
  Bottom 1.016: D201.A D202.C
N$12  (via drill 0.5)
  Top 0.61: RN201.6 65.09,94.28 63.82,93.01 v63.82,67.61
  Top 1.016: D209.A D201.C
  Bottom 1.016: D201.C 58.42,67.29 58.74,67.61 v63.82,67.61 82.55,67.61 90.49,75.55 93.66,75.55 94.61,76.5 X201.3
N$13  (via drill 0.5)
  Top 0.406: v13.65,79.67 v13.65,73.01
  Bottom 0.406: D101.AG v13.65,79.67 | v13.65,73.01 R103.2
N$15
  Bottom 1.016: D217.A D218.C
N$16
  Bottom 1.016: D225.C D226.A
N$17
  Top 0.61: RN201.8 58.42,93.01 D217.C
  Top 1.016: D225.A D217.C
  Bottom 1.016: D217.C 58.42,73.32 58.74,73.64 80.01,73.64 81.92,75.55 81.92,84.44 83.5,86.02 93.66,86.02 94.61,86.98 X201.1
N$18  (via drill 0.5)
  Top 0.61: v85.41,89.52 v85.41,83.8
  Top 1.016: D210.C D202.A D226.C D218.A
  Bottom 0.61: OK201.7 62.55,89.83 62.87,89.52 67.63,89.52 | 67.63,89.52 v85.41,89.52 | OK201.5 67.63,89.52
  Bottom 1.016: X201.2 v85.41,83.8 85.09,83.8 84.14,82.85 84.14,73.64 82.55,72.05 D218.A
N$19
  Bottom 1.016: D204.C D203.A
N$20
  Bottom 1.016: D210.A D209.C
N$21
  Bottom 1.016: D211.C D212.A
N$22  (via drill 0.5)
  Top 0.61: RN201.2 75.25,94.28 73.98,93.01 v73.98,55.54
  Top 1.016: D211.A D203.C
  Bottom 1.016: D203.C 58.42,54.91 59.05,55.54 v73.98,55.54 82.55,55.54 85.09,53 92.08,53 93.03,53.95 93.03,54.59 X202.3
N$31
  Bottom 1.016: D219.A D220.C
N$32
  Bottom 1.016: D227.C D228.A
N$33  (via drill 0.5)
  Top 0.61: RN201.4 70.17,94.28 68.9,93.01 v68.9,88.25 | v66.36,88.25 v66.36,61.57
  Top 1.016: D227.A D219.C
  Bottom 0.61: v68.9,88.25 v66.36,88.25
  Bottom 1.016: D219.C 58.42,61.26 58.74,61.57 v66.36,61.57 88.27,61.57 93.03,66.34 X202.1
N$34  (via drill 0.5)
  Top 0.61: OK201.3 v72.71,88.25 72.71,86.66 71.44,85.39 71.44,74.28 72.71,73.01 v72.71,59.99 | v77.79,88.25 OK201.1
  Top 1.016: D212.C D204.A D228.C D220.A
  Bottom 0.61: v72.71,88.25 v77.79,88.25 | D220.A v72.71,59.99
  Bottom 1.016: X202.2 93.03,61.26 91.76,59.99 D220.A
N$35
  Bottom 1.016: D205.A D206.C
N$36
  Bottom 1.016: D213.C D214.A
N$37  (via drill 0.5)
  Top 0.61: RN202.4 v70.8,22.52 | v63.5,22.52 63.5,38.4 62.55,39.35 D213.A
  Top 1.016: D213.A D205.C
  Bottom 0.61: v70.8,22.52 v63.5,22.52
  Bottom 1.016: D213.A 58.42,38.4 59.05,37.76 89.22,37.76 93.34,33.63 94.3,33.63 X203.3
N$39
  Bottom 1.016: D222.C D221.A
N$40
  Bottom 1.016: D229.C D230.A
N$41  (via drill 0.5)
  Top 0.61: RN202.2 75.88,19.03 74.3,20.62 v74.3,23.79 | v64.77,23.79 64.77,44.43 63.82,45.38 D229.A
  Top 1.016: D229.A D221.C
  Bottom 0.61: v74.3,23.79 v64.77,23.79
  Bottom 1.016: D229.A 58.42,44.43 59.05,43.79 82.87,43.79 86.68,47.6 93.34,47.6 94.61,46.33 X203.1
N$42
  Top 0.61: OK202.8 60.64,14.27 63.18,16.81 RN202.7
N$43
  Top 0.61: OK202.6 65.72,14.27 68.26,16.81 RN202.5
N$44
  Top 0.61: OK202.4 70.8,14.27 73.34,16.81 RN202.3
N$45
  Top 0.61: OK202.2 75.88,14.27 78.42,16.81 RN202.1
N$46
  Top 0.61: OK201.2 75.25,91.42 77.79,93.96 RN201.1
N$48
  Top 0.61: OK201.4 70.17,91.42 72.71,93.96 RN201.3
N$49  (via drill 0.5)
  Top 0.61: OK202.3 v73.34,11.73 | v78.42,11.73 OK202.1 | D214.C 81.92,39.35 82.55,38.71 v82.55,11.73
  Top 1.016: D214.C D206.A D230.C D222.A
  Bottom 0.61: v73.34,11.73 v78.42,11.73 v82.55,11.73
  Bottom 1.016: D214.C 94.3,39.35 X203.2
N$50
  Bottom 1.016: D207.A D208.C
N$51
  Bottom 1.016: D216.A D215.C
N$52
  Top 0.61: RN202.8 60.64,26.33 59.69,27.29 D215.A
  Top 1.016: D215.A D207.C
  Bottom 1.016: D215.A 65.72,27.29 67.31,25.7 80.01,25.7 81.28,24.43 81.28,17.12 82.55,15.86 88.27,15.86 92.71,11.41 X204.3
N$54
  Bottom 1.016: D223.A D224.C
N$55
  Bottom 1.016: D231.C D232.A
N$56  (via drill 0.5)
  Top 0.61: RN202.6 v65.72,21.25 | v62.23,21.25 62.23,32.36 61.28,33.32 D231.A
  Top 1.016: D231.A D223.C
  Bottom 0.61: v65.72,21.25 v62.23,21.25
  Bottom 1.016: D231.A 58.42,32.36 59.05,31.73 84.45,31.73 89.85,26.33 93.34,26.33 94.61,25.06 X204.1
N$57  (via drill 0.5)
  Top 0.61: OK202.7 v63.18,11.73 | v68.26,11.73 OK202.5 | D216.C v80.96,10.46
  Top 1.016: D224.A D232.C 80.96,32.05 80.96,31.41 D208.A D216.C
  Bottom 0.61: v63.18,11.73 v68.26,11.73 69.53,10.46 v80.96,10.46
  Bottom 1.016: D216.C 84.45,27.29 87,24.75 90.49,24.75 91.12,24.11 91.12,18.08 92.71,16.49 X204.2
N$64
  Top 0.61: OK201.6 65.09,91.42 67.63,93.96 RN201.5
N$65
  Top 0.61: OK201.8 60.01,91.42 62.55,93.96 RN201.7
O00  (via drill 0.5)
  Top 0.406: v83.82,87.61 83.82,71.42 v82.87,70.47 | v55.56,70.47 55.56,54.59 52.7,51.73 52.7,50.78 50.48,48.56 IC101.29
  Bottom 0.406: LED201.K v83.82,87.61 | v82.87,70.47 v55.56,70.47
O01  (via drill 0.5)
  Top 0.406: LED205.K 87.95,71.73 84.77,68.56 v84.77,64.75 | v56.52,64.75 56.52,54.27 55.24,53 v55.24,48.24 | v52.7,48.24 50.48,46.02 IC101.28
  Bottom 0.406: v84.77,64.75 v56.52,64.75 | v55.24,48.24 v52.7,48.24
O02  (via drill 0.5)
  Top 0.406: LED202.K 87,65.07 85.72,63.8 85.72,54.59 v83.5,52.37 | v56.52,52.37 v56.52,43.48
  Bottom 0.406: v83.5,52.37 v56.52,52.37 | v56.52,43.48 IC101.27
O03  (via drill 0.5)
  Top 0.406: LED206.K v87.95,49.83 | v53.98,49.83 v53.98,40.94
  Bottom 0.406: v87.95,49.83 v53.98,49.83 | v53.98,40.94 IC101.26
O04  (via drill 0.5)
  Top 0.406: v85.72,42.84 85.72,45.38 84.45,46.65 v83.19,46.65 | v55.24,46.65 v55.24,38.4
  Bottom 0.406: LED203.K v85.72,42.84 | v83.19,46.65 v55.24,46.65 | v55.24,38.4 IC101.25
O05  (via drill 0.5)
  Top 0.406: v85.72,32.68 v85.72,40.94 | v56.52,40.94 v56.52,35.86
  Bottom 0.406: LED207.K v85.72,32.68 | v85.72,40.94 v56.52,40.94 | v56.52,35.86 IC101.24
O06  (via drill 0.5)
  Top 0.406: v84.77,20.3 v84.77,34.59 | v56.52,34.59 v56.52,33.32
  Bottom 0.406: LED204.K v84.77,20.3 | v84.77,34.59 v56.52,34.59 | v56.52,33.32 IC101.23
O07  (via drill 0.5)
  Top 0.406: v83.82,10.14 v83.82,28.87
  Bottom 0.406: LED208.K v83.82,10.14 | v83.82,28.87 57.47,28.87 55.56,30.78 IC101.22
PLUGGED  (via drill 0.5)
  Top 0.406: v12.7,71.73 12.7,83.48 10.89,85.3 10.48,85.3 CON101.3
  Bottom 0.406: IC101.39 37.15,73.96 35.88,72.69 31.75,72.69 30.8,71.73 v12.7,71.73
Q-CLK
  Top 0.813: IC104.8 29.53,27.29 QG101.8 28.89,29.19 31.43,31.73 31.43,45.38 32.07,46.02 IC101.13
SCK  (via drill 0.5)
  Top 0.406: IC104.13 34.61,17.76 35.88,19.03 35.88,58.4 35.56,58.72 IC101.8 | IC103.6 42.23,7.28 41.27,8.24 v41.27,9.19
  Bottom 0.406: SV101.3 51.12,11.09 49.21,9.19 v41.27,9.19 34.29,9.19 33.34,10.14 33.34,14.59 IC104.13
SPG
  Bottom 0.406: R107.1 R106.2 53.02,82.53 48.9,78.4 IC101.40
V-NETZTEIL1
  Bottom 1.27: CON101.1 19.05,90.47 21.91,93.33 D103.A

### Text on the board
Bottom: MBCAN-Projekt | (c) Dr.-Ing. Th. Wiesner | 06.01.2024 | mbc88dc.brd | bottom
tNames: HW: 24.01.06 | +18V | DC | B | Status | (c) Dr.-Ing. Th. Wiesner | MBCAN-Projekt | B | IN | B | OUT | B | mbc-88-DC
